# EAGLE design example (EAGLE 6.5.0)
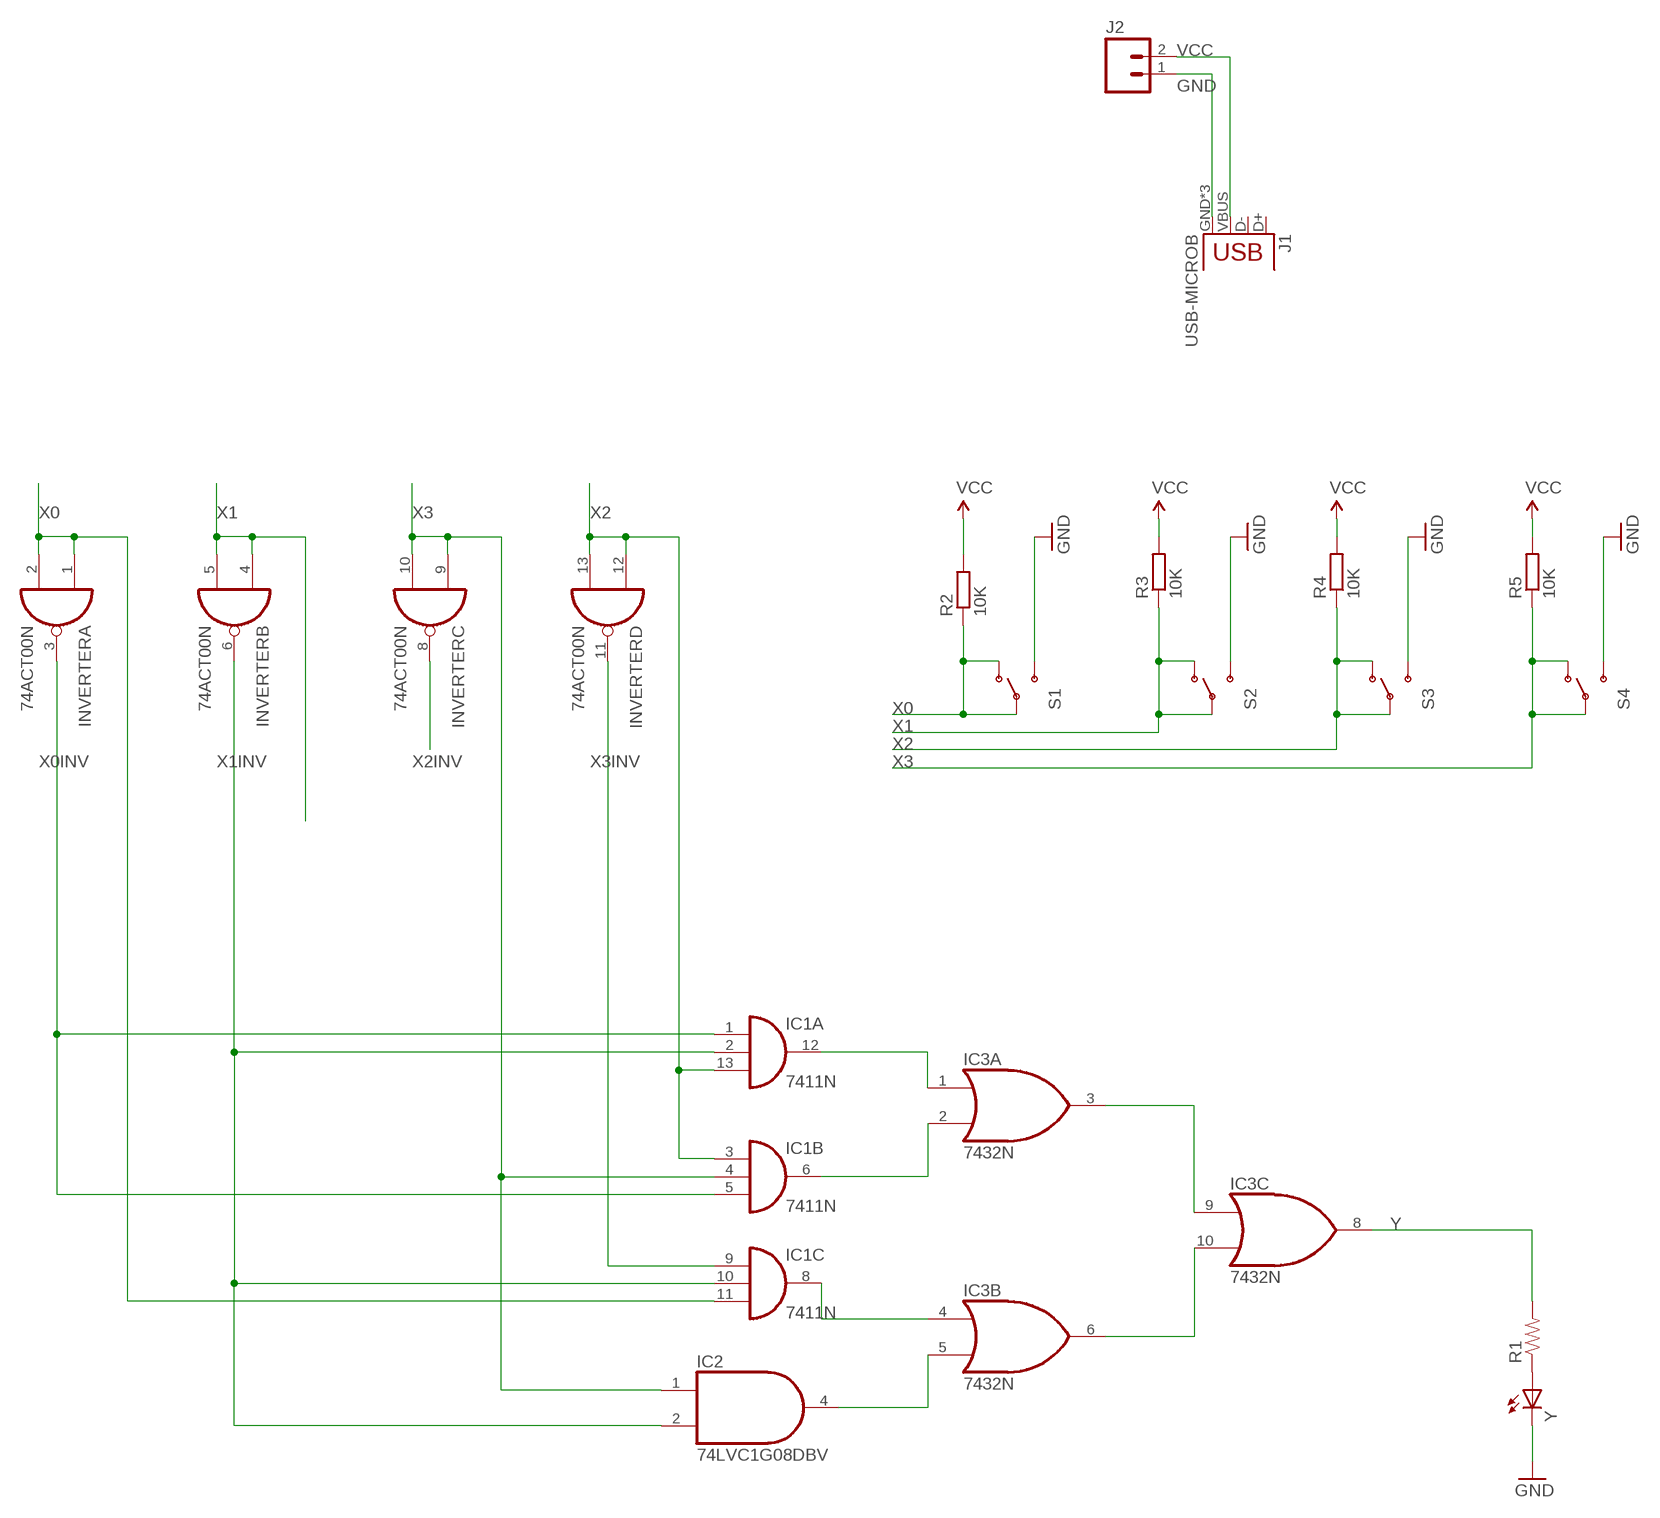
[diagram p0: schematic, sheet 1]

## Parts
IC1  7411N  [DIL14]
IC2  74LVC1G08DBV  [SOT23-5]
IC3  7432N  [DIL14]
INVERTER  74ACT00N  [DIL14]
J1  USB-MICROB  [USB-MICROB]
J2  M02PTH  [1X02]
R1  RESISTORPTH-1/4W  [AXIAL-0.4]
R2  10K  R-EU_R0805  [R0805]
R3  10K  R-EU_R0805  [R0805]
R4  10K  R-EU_R0805  [R0805]
R5  10K  R-EU_R0805  [R0805]
S1  SWITCH-SPDTPTH  [SWITCH-SPDT]
S2  SWITCH-SPDTPTH  [SWITCH-SPDT]
S3  SWITCH-SPDTPTH  [SWITCH-SPDT]
S4  SWITCH-SPDTPTH  [SWITCH-SPDT]
Y  LEDCHIPLED_0603  [CHIPLED_0603]

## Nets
GND: J1.GND J1.MT1(GND) J1.MT2(GND) J2.1 S1.3(S) S2.3(S) S3.3(S) S4.3(S) Y.C
N$1: IC1.12(A:O) IC3.1(A:I0)
N$2: IC1.6(B:O) IC3.2(A:I1)
N$3: IC1.8(C:O) IC3.4(B:I0)
N$4: IC2.4(O) IC3.5(B:I1)
N$5: IC3.3(A:O) IC3.9(C:I0)
N$6: IC3.6(B:O) IC3.10(C:I1)
N$7: R1.P$1 Y.A
VCC: J1.VBUS J2.2 R2.2 R3.2 R4.2 R5.2
X0: IC1.11(C:I2) INVERTER.1(A:I0) INVERTER.2(A:I1) R2.1 S1.1(O) S1.2(P)
X0INV: IC1.1(A:I0) IC1.5(B:I2) INVERTER.3(A:O)
X1: INVERTER.4(B:I0) INVERTER.5(B:I1) R3.1 S2.1(O) S2.2(P)
X1INV: IC1.2(A:I1) IC1.10(C:I1) IC2.2(I1) INVERTER.6(B:O)
X2: IC1.3(B:I0) IC1.13(A:I2) INVERTER.12(D:I0) INVERTER.13(D:I1) R4.1 S3.1(O) S3.2(P)
X2INV: INVERTER.8(C:O)
X3: IC1.4(B:I1) IC2.1(I0) INVERTER.9(C:I0) INVERTER.10(C:I1) R5.1 S4.1(O) S4.2(P)
X3INV: IC1.9(C:I0) INVERTER.11(D:O)
Y: IC3.8(C:O) R1.P$2
Unconnected: IC3.11(D:O) IC3.12(D:I0) IC3.13(D:I1) J1.D+ J1.D-

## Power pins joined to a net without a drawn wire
GND: IC1.7(P:GND) IC2.3(GND) IC3.7(P:GND) INVERTER.7(P:GND)
VCC: IC1.14(P:VCC) IC2.5(VCC) IC3.14(P:VCC) INVERTER.14(P:VCC)

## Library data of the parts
IC1 = example_function:74*11: Triple 3-input AND gate
IC2 = 74xx-little-us:74*1G08: 2-input AND gate
IC3 = 74xx-us:74*32: Quad 2-input OR gate
INVERTER = 74xx-eu:74*00: Quad 2-input NAND gate
J1 = SparkFun-Connectors:USB: USB Connectors USB-B-PTH is fully proven SKU : PRT-00139/CONN-08278 USB-miniB is fully proven SKU : PRT-00587 USB-A-PCB is untested. USB-A-H is throughly reviewed, but untested. Spark Fun Electronics SKU : PRT-00437 USB-B-SMT is throughly reviewed, but untested. Needs silkscreen touching up.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; PROD_ID: CONN-09505
J2 = SparkFun-Connectors:M02: Standard 2-pin 0.1" header. Use with
R1 = SparkFun-Passives:RESISTOR: Resistor
R2-R5 = resistor:R-EU_: RESISTOR, European symbol
S1-S4 = SparkFun-Electromechanical:SWITCH-SPDT: SPDT Switch Simple slide switch, Spark Fun Electronics SKU : COM-00102 DPDT SMT slide switch, AYZ0202, SWCH-08179; PROD_ID: SWCH-08261
Y = led:LED: LED

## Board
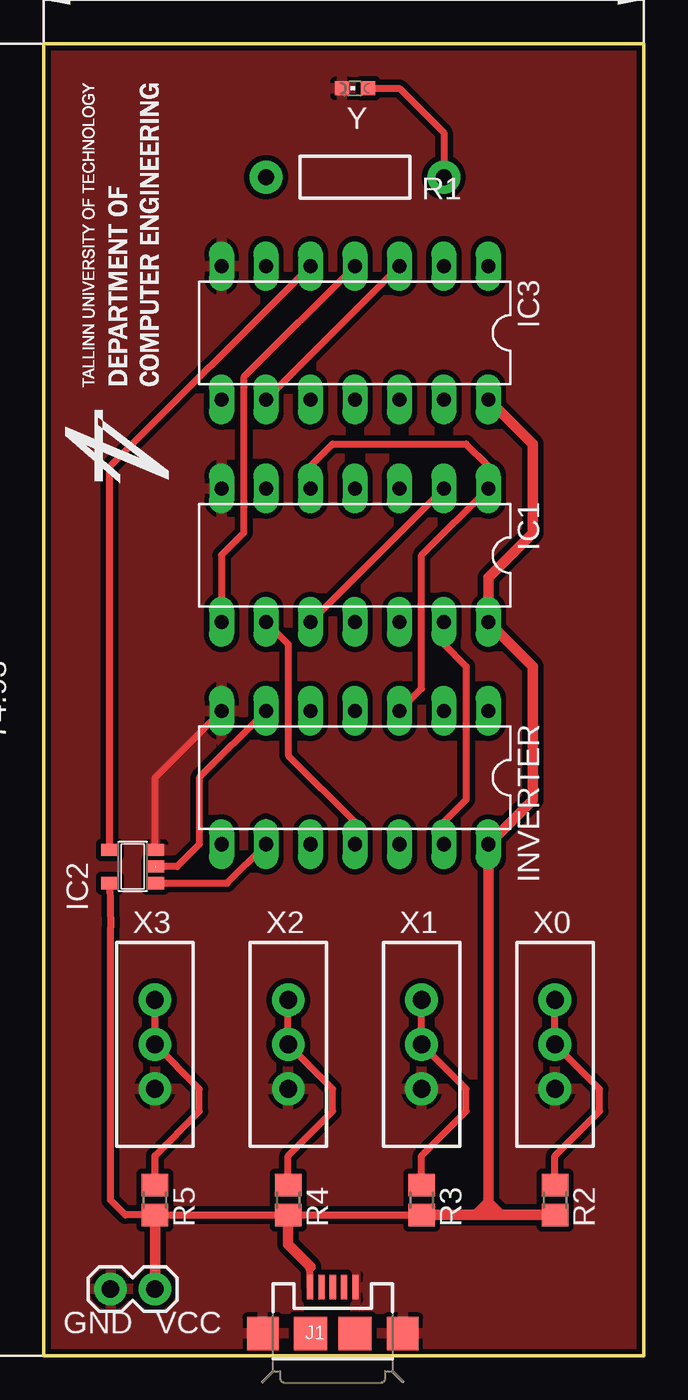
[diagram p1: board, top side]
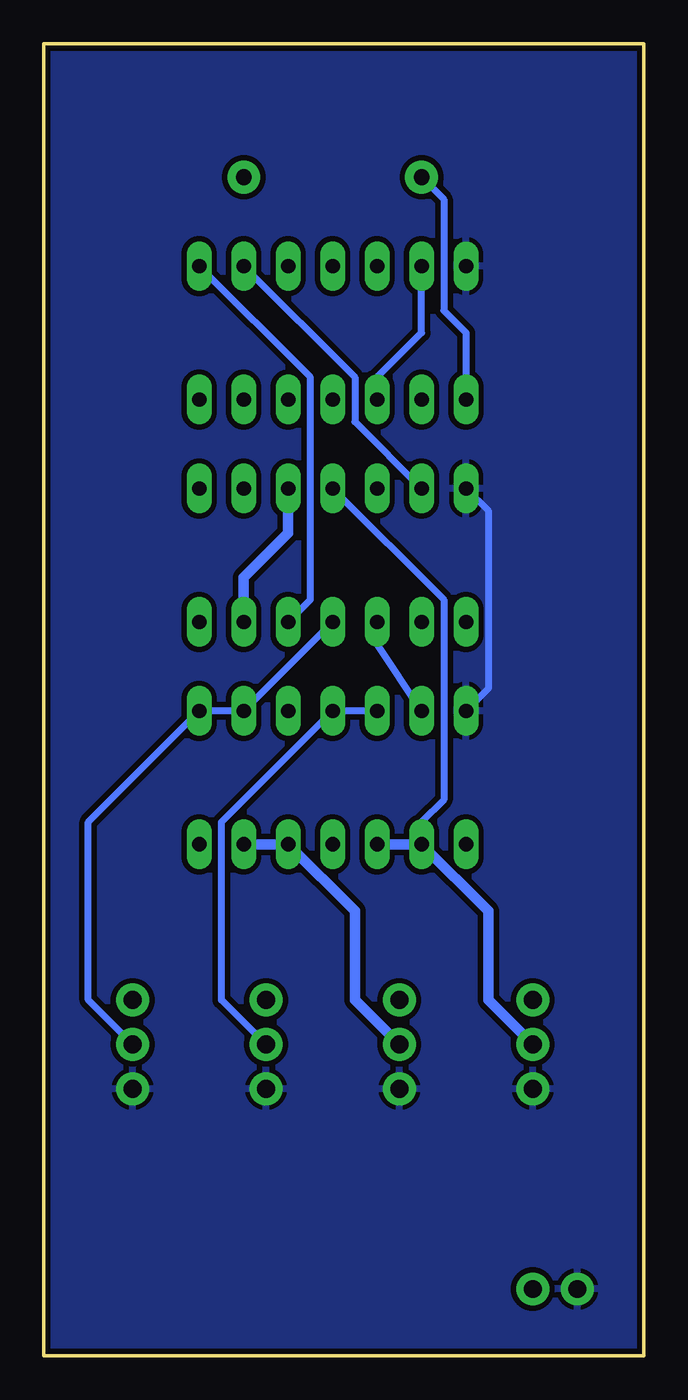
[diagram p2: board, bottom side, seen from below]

Size 34.29 x 74.93 mm. Coordinates in mm from the lower left corner, seen from the top.
Outline: 0,74.93 0,0 34.29,0 34.29,74.93 0,74.93
Copper layers (1*16): Top 0.035mm / dielectric 1.5mm / Bottom 0.035mm
Design rules "SparkFun": minimum track width 8mil, minimum drill 20mil, track to track 8mil, track to pad 8mil, pad to pad 8mil, via to via 8mil, smd to smd 8mil, copper to edge 8mil, drill to drill 8mil, minimum pad ring 12mil, minimum via ring 10mil, stop-mask expansion 4mil, vias tented up to drill 20mil, thermal gap 10mil

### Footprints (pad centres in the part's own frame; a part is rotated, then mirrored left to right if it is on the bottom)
DIL14 = drill 0.813 long: 1 -7.62,-3.81; 2 -5.08,-3.81; 3 -2.54,-3.81; 4 0,-3.81; 5 2.54,-3.81; 6 5.08,-3.81; 7 7.62,-3.81; 8 7.62,3.81; 9 5.08,3.81; 10 2.54,3.81; 11 0,3.81; 12 -2.54,3.81; 13 -5.08,3.81; 14 -7.62,3.81
SOT23-5 = smd 0.69 x 0.99: 1 -0.95,-1.29; 2 0,-1.29; 3 0.95,-1.29; 4 0.95,1.3; 5 -0.95,1.3
USB-MICROB = smd 0.35 x 1.4: D+ 0,2.65; D- -0.65,2.65; GND 1.3,2.65; ID 0.65,2.65; VBUS -1.3,2.65 | smd 1.8 x 1.9: MT1 -4,0; MT2 4,0 | smd 1.9 x 1.9: P$1 -1.27,0; P$2 1.27,0
1X02 = drill 1.016 pad 1.88: 1 0,0; 2 2.54,0
AXIAL-0.4 = drill 0.9 pad 1.88: P$1 -5.08,0; P$2 5.08,0
R0805 = smd 1.3 x 1.5: 1 -0.85,0; 2 0.85,0
SWITCH-SPDT = drill 1.016 pad 1.88: 1 0,2.54; 2 0,0; 3 0,-2.54
CHIPLED_0603 = smd 0.8 x 0.8: A 0,-0.75; C 0,0.75

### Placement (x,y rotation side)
IC1  17.78,45.72 180 top
IC2  5.08,27.94 90 top
IC3  17.78,58.42 180 top
INVERTER  17.78,33.02 180 top
J1  16.51,1.27 0 top
J2  3.81,3.81 0 top
R1  17.78,67.31 180 top
R2  29.21,8.89 270 top
R3  21.59,8.89 270 top
R4  13.97,8.89 270 top
R5  6.35,8.89 270 top
S1  29.21,17.78 0 top
S2  21.59,17.78 0 top
S3  13.97,17.78 0 top
S4  6.35,17.78 0 top
Y  17.78,72.39 90 top

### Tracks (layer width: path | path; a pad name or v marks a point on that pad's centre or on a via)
GND
  Top 0.406: IC2.3 6.37,33.04 INVERTER.7
  Bottom 0.406: IC1.7 8.89,48.26 8.89,38.1 INVERTER.7
  pour Top (isolate 0.305): 0,74.93 34.29,74.93 34.29,0 0,0
  pour Bottom (isolate 0.305): 0,74.93 34.29,74.93 34.29,0 0,0
N$1
  Bottom 0.406: IC1.12 19.05,43.18 19.05,55.88 IC3.1
N$2
  Bottom 0.406: IC3.2 16.51,55.88 16.51,53.34 IC1.6
N$3
  Top 0.406: IC3.4 11.43,55.88 11.43,46.99 10.16,45.72 IC1.8
N$4
  Top 0.406: IC2.4 3.78,50.77 IC3.5
N$5
  Top 0.406: IC3.3 IC3.9
N$6
  Bottom 0.406: IC3.10 15.24,55.88 12.7,58.42 IC3.6
N$7
  Top 0.406: Y.A 20.32,72.39 22.86,69.85 R1.P$1
VCC
  Top 0.406: IC2.5 3.81,24.42 3.81,8.89 4.66,8.04 R5.2 R4.2 R3.2 | J1.VBUS 15.21,5.05
  Top 0.61: 25.4,8.76 INVERTER.14 27.94,31.75 27.94,39.37 IC1.14 25.4,44.45 27.94,46.99 27.94,52.07 IC3.14 | 25.4,8.76 25.4,8.04 R2.2 R3.2 | 25.4,8.76 26.04,8.13 | 25.4,8.76 24.76,8.13 | R4.2 13.97,6.35 15.24,5.08 15.21,5.05 | J2.2 R5.2
X0
  Top 0.406: S1.1 S1.2 31.75,15.24 31.75,13.97 29.21,11.43 R2.1
  Bottom 0.406: S1.2 31.75,20.32 31.75,30.48 INVERTER.1 INVERTER.2 IC1.11
X0INV
  Top 0.406: INVERTER.3 21.59,38.1 21.59,45.72 IC1.1 25.4,50.8 24.13,52.07 16.51,52.07 15.24,50.8 IC1.5
X1
  Top 0.406: S2.1 S2.2 24.13,15.24 24.13,13.97 21.59,11.43 R3.1
  Bottom 0.406: S2.2 24.13,20.32 24.13,30.48 INVERTER.4 INVERTER.5
X1INV
  Top 0.406: IC1.2 IC1.10 | INVERTER.6 8.89,33.02 8.89,29.21 7.62,27.94 IC2.2
  Bottom 0.406: INVERTER.6 15.24,40.64 IC1.10
X2
  Top 0.406: IC1.13 22.86,40.64 24.13,39.37 24.13,31.75 22.86,30.48 INVERTER.13 | S3.1 S3.2 16.51,15.24 16.51,13.97 13.97,11.43 R4.1
  Bottom 0.61: S3.2 16.51,20.32 16.51,25.4 INVERTER.12 INVERTER.13 | IC1.3 20.32,46.99 22.86,44.45 IC1.13
X3
  Top 0.406: 12.7,30.48 INVERTER.9 10.48,26.99 IC2.1 | S4.1 S4.2 8.89,15.24 8.89,13.97 6.35,11.43 R5.1
  Bottom 0.406: IC1.4 11.43,43.18 11.43,31.75 12.7,30.48 INVERTER.9
  Bottom 0.61: INVERTER.10 INVERTER.9 8.89,25.4 8.89,20.32 S4.2
X3INV
  Top 0.406: IC1.9 13.97,40.64 13.97,34.29 17.78,30.48 INVERTER.11
Y
  Bottom 0.406: R1.P$2 11.43,66.04 11.43,59.69 10.16,58.42 IC3.8

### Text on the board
tPlace: R1 | C:/Users/keijo/Dropbox/Digitaalsüsteemid/Eagle/ATI_logo_bitmap.bmp | X3 | X2 | X1 | X0 | GND | VCC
